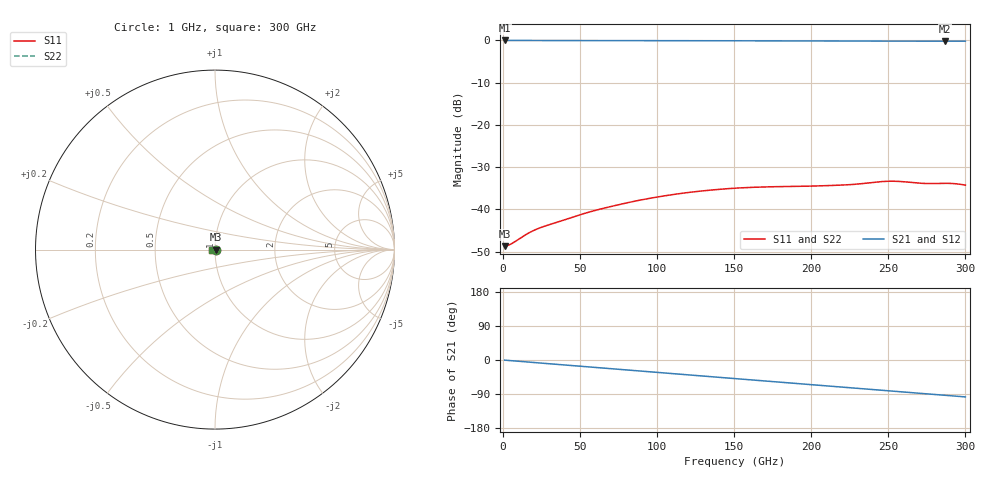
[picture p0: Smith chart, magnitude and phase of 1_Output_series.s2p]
#  Hz  S  RI  R  50
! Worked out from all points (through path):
!   300 points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, 1 GHz to 300 GHz, reference 50 ohm
!   highest |S21| = -0.03 dB at 1 GHz (marker M1); lowest = -0.2 dB at 287 GHz (marker M2)
!   group delay of S21, straight-line fit = 902 fs
!   lowest |S11| = -48.7 dB at 1 GHz (marker M3), VSWR 1.01, Z = 50.4 + j0.00391 ohm
!   |S11| at or under -10 dB: start of sweep to end of sweep
!   |S22| runs from -48.7 to -33.3 dB; largest |S21 - S12| = 0.00052
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1e9  0.00366 3.88e-05  0.9965 -0.00591  0.9964 -0.0059  0.00369 3.3e-05
3e9  0.00373 0.000106  0.9962 -0.0177  0.9962 -0.0177  0.00376 8.98e-05
6e9  0.00396 0.000147  0.9954 -0.0353  0.9954 -0.0353  0.00397 0.00012
1.5e10  0.00502 -0.000481  0.9909 -0.0869  0.9909 -0.0869  0.005 -0.000483
2.2e10  0.00562 -0.00162  0.986 -0.1262  0.986 -0.1262  0.00561 -0.00159
2.9e10  0.00582 -0.00287  0.9799 -0.1654  0.9798 -0.1654  0.00584 -0.00286
5.1e10  0.00555 -0.00674  0.9501 -0.2859  0.95 -0.2859  0.00554 -0.00673
6.1e10  0.00489 -0.00853  0.9319 -0.3392  0.9319 -0.3391  0.00491 -0.00853
7.3e10  0.00379 -0.0105  0.906 -0.4015  0.906 -0.4016  0.00378 -0.0105
8.7e10  0.00214 -0.0125  0.8708 -0.4718  0.8707 -0.4717  0.00214 -0.0125
1.01e11  0.000145 -0.0141  0.83 -0.539  0.8301 -0.539  0.000145 -0.0141
1.24e11  -0.00354 -0.0157  0.7522 -0.6418  0.7522 -0.6418  -0.00353 -0.0157
1.51e11  -0.0078 -0.016  0.6446 -0.7483  0.6446 -0.7483  -0.0078 -0.016
1.77e11  -0.011 -0.0149  0.5264 -0.8339  0.5263 -0.8339  -0.011 -0.0149
2.01e11  -0.0128 -0.0138  0.4069 -0.8957  0.4068 -0.8957  -0.0128 -0.0138
2.25e11  -0.0144 -0.0132  0.2809 -0.9395  0.2809 -0.9396  -0.0144 -0.0132
2.51e11  -0.0179 -0.0119  0.1422 -0.9675  0.1423 -0.9676  -0.0179 -0.0119
2.58e11  -0.0185 -0.0106  0.1044 -0.9723  0.1043 -0.9725  -0.0185 -0.0106
2.74e11  -0.0183 -0.00849  0.0159 -0.9772  0.0161 -0.977  -0.0183 -0.00847
2.87e11  -0.0189 -0.0073  -0.0545 -0.9745  -0.0546 -0.9749  -0.019 -0.00733
2.94e11  -0.0191 -0.00596  -0.0924 -0.9721  -0.0928 -0.972  -0.0192 -0.00596
3e11  -0.0187 -0.0047  -0.1256 -0.9688  -0.1256 -0.9683  -0.0187 -0.00466
